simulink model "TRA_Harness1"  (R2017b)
settings: Solver=FixedStepDiscrete  StartTime=0.0  StopTime=16  FixedStep=0.01  RelTol=1e-3  EnableMultiTasking=on
undefined symbols (not defined in the file): sigbuilder_block
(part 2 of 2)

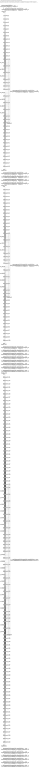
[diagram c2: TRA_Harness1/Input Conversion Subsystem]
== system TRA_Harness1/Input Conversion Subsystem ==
  note: This subsystem has been inserted by Simulink to adapt the output of the source blocks to the interface required by the harnessed component. Modifying the contents of this subsystem may result in compilation and simulation failure.
  Inport_1 : Inport
  Inport_2 : Inport  Port=2
  Inport_3 : Inport  Port=3
  Inport_4 : Inport  Port=4
  Inport_5 : Inport  Port=5
  Inport_6 : Inport  Port=6
  Inport_7 : Inport  Port=7
  Inport_8 : Inport  Port=8
  Inport_9 : Inport  Port=9
  Inport_10 : Inport  Port=10
  Inport_11 : Inport  Port=11
  Inport_12 : Inport  Port=12
  Inport_13 : Inport  Port=13
  Inport_14 : Inport  Port=14
  Inport_15 : Inport  Port=15
  Inport_16 : Inport  Port=16
  Inport_17 : Inport  Port=17
  Inport_18 : Inport  Port=18
  Inport_19 : Inport  Port=19
  Inport_20 : Inport  Port=20
  Inport_21 : Inport  Port=21
  Inport_22 : Inport  Port=22
  Inport_23 : Inport  Port=23
  Inport_24 : Inport  Port=24
  Inport_25 : Inport  Port=25
  Inport_26 : Inport  Port=26
  Inport_27 : Inport  Port=27
  Inport_28 : Inport  Port=28
  Inport_29 : Inport  Port=29
  Inport_30 : Inport  Port=30
  Inport_31 : Inport  Port=31
  Inport_32 : Inport  Port=32
  Inport_33 : Inport  Port=33
  Inport_34 : Inport  Port=34
  Inport_35 : Inport  Port=35
  Inport_36 : Inport  Port=36
  Inport_37 : Inport  Port=37
  Inport_38 : Inport  Port=38
  Inport_39 : Inport  Port=39
  Inport_40 : Inport  Port=40
  Inport_41 : Inport  Port=41
  Inport_42 : Inport  Port=42
  Inport_43 : Inport  Port=43
  Inport_44 : Inport  Port=44
  Inport_45 : Inport  Port=45
  Inport_46 : Inport  Port=46
  Inport_47 : Inport  Port=47
  Inport_48 : Inport  Port=48
  Inport_49 : Inport  Port=49
  Inport_50 : Inport  Port=50
  Inport_51 : Inport  Port=51
  Inport_52 : Inport  Port=52
  Inport_53 : Inport  Port=53
  Inport_54 : Inport  Port=54
  Inport_55 : Inport  Port=55
  Inport_56 : Inport  Port=56
  Inport_57 : Inport  Port=57
  Inport_58 : Inport  Port=58
  Inport_59 : Inport  Port=59
  Inport_60 : Inport  Port=60
  Inport_61 : Inport  Port=61
  Inport_62 : Inport  Port=62
  Inport_63 : Inport  Port=63
  Inport_64 : Inport  Port=64
  Inport_65 : Inport  Port=65
  Inport_66 : Inport  Port=66
  Inport_67 : Inport  Port=67
  Inport_68 : Inport  Port=68
  Inport_69 : Inport  Port=69
  Inport_70 : Inport  Port=70
  Inport_71 : Inport  Port=71
  Inport_72 : Inport  Port=72
  Inport_73 : Inport  Port=73
  Inport_74 : Inport  Port=74
  Inport_75 : Inport  Port=75
  Inport_76 : Inport  Port=76
  Inport_77 : Inport  Port=77
  Inport_78 : Inport  Port=78
  Inport_79 : Inport  Port=79
  Inport_80 : Inport  Port=80
  Inport_81 : Inport  Port=81
  Inport_82 : Inport  Port=82
  Inport_83 : Inport  Port=83
  Inport_84 : Inport  Port=84
  Inport_85 : Inport  Port=85
  Inport_86 : Inport  Port=86
  Inport_87 : Inport  Port=87
  Inport_88 : Inport  Port=88
  Inport_89 : Inport  Port=89
  Inport_90 : Inport  Port=90
  Inport_91 : Inport  Port=91
  Inport_92 : Inport  Port=92
  Inport_93 : Inport  Port=93
  Inport_94 : Inport  Port=94
  Inport_95 : Inport  Port=95
  Inport_96 : Inport  Port=96
  Inport_97 : Inport  Port=97
  Inport_98 : Inport  Port=98
  Inport_99 : Inport  Port=99
  Inport_100 : Inport  Port=100
  Inport_101 : Inport  Port=101
  Inport_102 : Inport  Port=102
  Inport_103 : Inport  Port=103
  Inport_104 : Inport  Port=104
  Inport_105 : Inport  Port=105
  Inport_106 : Inport  Port=106
  Inport_107 : Inport  Port=107
  Inport_108 : Inport  Port=108
  Inport_109 : Inport  Port=109
  Inport_110 : Inport  Port=110
  Inport_111 : Inport  Port=111
  Inport_112 : Inport  Port=112
  Inport_113 : Inport  Port=113
  Inport_114 : Inport  Port=114
  Inport_115 : Inport  Port=115
  Inport_116 : Inport  Port=116
  Inport_117 : Inport  Port=117
  Inport_118 : Inport  Port=118
  Inport_119 : Inport  Port=119
  Inport_120 : Inport  Port=120
  Inport_121 : Inport  Port=121
  Inport_122 : Inport  Port=122
  Inport_123 : Inport  Port=123
  Inport_124 : Inport  Port=124
  Inport_125 : Inport  Port=125
  Inport_126 : Inport  Port=126
  Inport_127 : Inport  Port=127
  Inport_128 : Inport  Port=128
  Inport_129 : Inport  Port=129
  Inport_130 : Inport  Port=130
  Inport_131 : Inport  Port=131
  Inport_132 : Inport  Port=132
  Inport_133 : Inport  Port=133
  Inport_134 : Inport  Port=134
  Inport_135 : Inport  Port=135
  Inport_136 : Inport  Port=136
  Inport_137 : Inport  Port=137
  Inport_138 : Inport  Port=138
  Inport_139 : Inport  Port=139
  Inport_140 : Inport  Port=140
  Inport_141 : Inport  Port=141
  Inport_142 : Inport  Port=142
  Inport_143 : Inport  Port=143
  Inport_144 : Inport  Port=144
  Inport_145 : Inport  Port=145
  Inport_146 : Inport  Port=146
  Inport_147 : Inport  Port=147
  Inport_148 : Inport  Port=148
  Inport_149 : Inport  Port=149
  Inport_150 : Inport  Port=150
  Inport_151 : Inport  Port=151
  Inport_152 : Inport  Port=152
  Inport_153 : Inport  Port=153
  Inport_154 : Inport  Port=154
  Inport_155 : Inport  Port=155
  Inport_156 : Inport  Port=156
  Inport_157 : Inport  Port=157
  Inport_158 : Inport  Port=158
  Inport_159 : Inport  Port=159
  Inport_160 : Inport  Port=160
  Inport_161 : Inport  Port=161
  Inport_162 : Inport  Port=162
  Inport_163 : Inport  Port=163
  Inport_164 : Inport  Port=164
  Inport_165 : Inport  Port=165
  Inport_166 : Inport  Port=166
  Inport_167 : Inport  Port=167
  Inport_168 : Inport  Port=168
  Inport_169 : Inport  Port=169
  Inport_170 : Inport  Port=170
  Inport_171 : Inport  Port=171
  Inport_172 : Inport  Port=172
  Inport_173 : Inport  Port=173
  Inport_174 : Inport  Port=174
  Inport_175 : Inport  Port=175
  Inport_176 : Inport  Port=176
  Inport_177 : Inport  Port=177
  Inport_178 : Inport  Port=178
  Inport_179 : Inport  Port=179
  Inport_180 : Inport  Port=180
  Inport_181 : Inport  Port=181
  Inport_182 : Inport  Port=182
  Inport_183 : Inport  Port=183
  Inport_184 : Inport  Port=184
  Inport_185 : Inport  Port=185
  Inport_186 : Inport  Port=186
  Inport_187 : Inport  Port=187
  Inport_188 : Inport  Port=188
  Inport_189 : Inport  Port=189
  Inport_190 : Inport  Port=190
  Inport_191 : Inport  Port=191
  Inport_192 : Inport  Port=192
  Inport_193 : Inport  Port=193
  Inport_194 : Inport  Port=194
  Inport_195 : Inport  Port=195
  Inport_196 : Inport  Port=196
  Inport_197 : Inport  Port=197
  Inport_198 : Inport  Port=198
  Inport_199 : Inport  Port=199
  Inport_200 : Inport  Port=200
  Inport_201 : Inport  Port=201
  Inport_202 : Inport  Port=202
  Inport_203 : Inport  Port=203
  Inport_204 : Inport  Port=204
  Inport_205 : Inport  Port=205
  Inport_206 : Inport  Port=206
  Inport_207 : Inport  Port=207
  Inport_208 : Inport  Port=208
  Inport_209 : Inport  Port=209
  Inport_210 : Inport  Port=210
  Inport_211 : Inport  Port=211
  Inport_212 : Inport  Port=212
  Inport_213 : Inport  Port=213
  Inport_214 : Inport  Port=214
  Inport_215 : Inport  Port=215
  Inport_216 : Inport  Port=216
  Inport_217 : Inport  Port=217
  Inport_218 : Inport  Port=218
  Inport_219 : Inport  Port=219
  Inport_220 : Inport  Port=220
  Inport_221 : Inport  Port=221
  Inport_222 : Inport  Port=222
  Inport_223 : Inport  Port=223
  Inport_224 : Inport  Port=224
  Inport_225 : Inport  Port=225
  Inport_226 : Inport  Port=226
  Inport_227 : Inport  Port=227
  Concat_1 : Concatenate  NumInputs=48
  Concat_2 : Concatenate  NumInputs=48
  Concat_3 : Concatenate  NumInputs=112
  Data_Conversion_{1..2,4,6..8,24} (7 alike) : DataTypeConversion  OutDataTypeStr=single
  Data_Conversion_{5,10..11,20,23} (5 alike) : DataTypeConversion  OutDataTypeStr=uint8
  Data_Conversion_{12,14..17,21} (6 alike) : DataTypeConversion  OutDataTypeStr=boolean
  Data_Conversion_13 : DataTypeConversion  OutDataTypeStr=uint32
  Data_Conversion_18 : DataTypeConversion  OutDataTypeStr=uint16
  Data_Conversion_19 : Reshape  OutputDimensionality=Customize  OutputDimensions=[112]
  Data_Conversion_22 : DataTypeConversion  OutDataTypeStr=uint16
  Data_Conversion_25 : DataTypeConversion  OutDataTypeStr=uint16
  Data_Conversion_3 : Reshape  OutputDimensionality=Customize  OutputDimensions=[48]
  Data_Conversion_9 : Reshape  OutputDimensionality=Customize  OutputDimensions=[48]
  RateTs_{1..22} (22 alike) : RateTransition
  SigSpec_1 : SignalSpecification
  SigSpec_10 : SignalSpecification  OutDataTypeStr=uint8  Unit=enum  Dimensions=[1]
  SigSpec_{11,13..16,19} (6 alike) : SignalSpecification  OutDataTypeStr=boolean  Unit=flag  Dimensions=[1]
  SigSpec_12 : SignalSpecification  OutDataTypeStr=uint32  Unit=min  Dimensions=[1]
  SigSpec_17 : SignalSpecification  OutDataTypeStr=uint16  Unit=mV  Dimensions=[112]
  SigSpec_18 : SignalSpecification  OutDataTypeStr=uint8  Unit=enum  Dimensions=[1]
  SigSpec_{2,4,6..7} (4 alike) : SignalSpecification  OutDataTypeStr=single  Unit=C  Dimensions=[1]
  SigSpec_20 : SignalSpecification  OutDataTypeStr=uint16  Unit=mV  Dimensions=[1]
  SigSpec_21 : SignalSpecification  OutDataTypeStr=uint8  Unit=numb  Dimensions=[1]
  SigSpec_22 : SignalSpecification  OutDataTypeStr=single  Unit=A  Dimensions=[1]
  SigSpec_23 : SignalSpecification  OutDataTypeStr=uint16  Unit=enum  Dimensions=[1]
  SigSpec_3 : SignalSpecification  OutDataTypeStr=single  Unit=C  Dimensions=[48]
  SigSpec_5 : SignalSpecification  OutDataTypeStr=uint8  Unit=numb  Dimensions=[1]
  SigSpec_8 : SignalSpecification  OutDataTypeStr=single  Unit=C  Dimensions=[48]
  SigSpec_9 : SignalSpecification  OutDataTypeStr=uint8  Unit=numb  Dimensions=[1]
  Outport_1 : Outport
  Outport_2 : Outport  Port=2
  Outport_3 : Outport  Port=3
  Outport_4 : Outport  Port=4
  Outport_5 : Outport  Port=5
  Outport_6 : Outport  Port=6
  Outport_7 : Outport  Port=7
  Outport_8 : Outport  Port=8
  Outport_9 : Outport  Port=9
  Outport_10 : Outport  Port=10
  Outport_11 : Outport  Port=11
  Outport_12 : Outport  Port=12
  Outport_13 : Outport  Port=13
  Outport_14 : Outport  Port=14
  Outport_15 : Outport  Port=15
  Outport_16 : Outport  Port=16
  Outport_17 : Outport  Port=17
  Outport_18 : Outport  Port=18
  Outport_19 : Outport  Port=19
  Outport_20 : Outport  Port=20
  Outport_21 : Outport  Port=21
  Outport_22 : Outport  Port=22
  Outport_23 : Outport  Port=23
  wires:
  SigSpec_1/1 -> Outport_1/1
  [send_fcn1] -> SigSpec_1/1
  SigSpec_2/1 -> Outport_2/1
  RateTs_1/1 -> SigSpec_2/1
  Data_Conversion_1/1 -> RateTs_1/1
  Inport_1/1 -> Data_Conversion_1/1
  SigSpec_3/1 -> Outport_3/1
  RateTs_2/1 -> SigSpec_3/1
  Data_Conversion_2/1 -> RateTs_2/1
  Data_Conversion_3/1 -> Data_Conversion_2/1
  Concat_1/1 -> Data_Conversion_3/1
  Inport_2/1 -> Concat_1/1
  Inport_3/1 -> Concat_1/2
  Inport_4/1 -> Concat_1/3
  Inport_5/1 -> Concat_1/4
  Inport_6/1 -> Concat_1/5
  Inport_7/1 -> Concat_1/6
  Inport_8/1 -> Concat_1/7
  Inport_9/1 -> Concat_1/8
  Inport_10/1 -> Concat_1/9
  Inport_11/1 -> Concat_1/10
  Inport_12/1 -> Concat_1/11
  Inport_13/1 -> Concat_1/12
  Inport_14/1 -> Concat_1/13
  Inport_15/1 -> Concat_1/14
  Inport_16/1 -> Concat_1/15
  Inport_17/1 -> Concat_1/16
  Inport_18/1 -> Concat_1/17
  Inport_19/1 -> Concat_1/18
  Inport_20/1 -> Concat_1/19
  Inport_21/1 -> Concat_1/20
  Inport_22/1 -> Concat_1/21
  Inport_23/1 -> Concat_1/22
  Inport_24/1 -> Concat_1/23
  Inport_25/1 -> Concat_1/24
  Inport_26/1 -> Concat_1/25
  Inport_27/1 -> Concat_1/26
  Inport_28/1 -> Concat_1/27
  Inport_29/1 -> Concat_1/28
  Inport_30/1 -> Concat_1/29
  Inport_31/1 -> Concat_1/30
  Inport_32/1 -> Concat_1/31
  Inport_33/1 -> Concat_1/32
  Inport_34/1 -> Concat_1/33
  Inport_35/1 -> Concat_1/34
  Inport_36/1 -> Concat_1/35
  Inport_37/1 -> Concat_1/36
  Inport_38/1 -> Concat_1/37
  Inport_39/1 -> Concat_1/38
  Inport_40/1 -> Concat_1/39
  Inport_41/1 -> Concat_1/40
  Inport_42/1 -> Concat_1/41
  Inport_43/1 -> Concat_1/42
  Inport_44/1 -> Concat_1/43
  Inport_45/1 -> Concat_1/44
  Inport_46/1 -> Concat_1/45
  Inport_47/1 -> Concat_1/46
  Inport_48/1 -> Concat_1/47
  Inport_49/1 -> Concat_1/48
  SigSpec_4/1 -> Outport_4/1
  RateTs_3/1 -> SigSpec_4/1
  Data_Conversion_4/1 -> RateTs_3/1
  Inport_50/1 -> Data_Conversion_4/1
  SigSpec_5/1 -> Outport_5/1
  RateTs_4/1 -> SigSpec_5/1
  Data_Conversion_5/1 -> RateTs_4/1
  Inport_51/1 -> Data_Conversion_5/1
  SigSpec_6/1 -> Outport_6/1
  RateTs_5/1 -> SigSpec_6/1
  Data_Conversion_6/1 -> RateTs_5/1
  Inport_52/1 -> Data_Conversion_6/1
  SigSpec_7/1 -> Outport_7/1
  RateTs_6/1 -> SigSpec_7/1
  Data_Conversion_7/1 -> RateTs_6/1
  Inport_53/1 -> Data_Conversion_7/1
  SigSpec_8/1 -> Outport_8/1
  RateTs_7/1 -> SigSpec_8/1
  Data_Conversion_8/1 -> RateTs_7/1
  Data_Conversion_9/1 -> Data_Conversion_8/1
  Concat_2/1 -> Data_Conversion_9/1
  Inport_54/1 -> Concat_2/1
  Inport_55/1 -> Concat_2/2
  Inport_56/1 -> Concat_2/3
  Inport_57/1 -> Concat_2/4
  Inport_58/1 -> Concat_2/5
  Inport_59/1 -> Concat_2/6
  Inport_60/1 -> Concat_2/7
  Inport_61/1 -> Concat_2/8
  Inport_62/1 -> Concat_2/9
  Inport_63/1 -> Concat_2/10
  Inport_64/1 -> Concat_2/11
  Inport_65/1 -> Concat_2/12
  Inport_66/1 -> Concat_2/13
  Inport_67/1 -> Concat_2/14
  Inport_68/1 -> Concat_2/15
  Inport_69/1 -> Concat_2/16
  Inport_70/1 -> Concat_2/17
  Inport_71/1 -> Concat_2/18
  Inport_72/1 -> Concat_2/19
  Inport_73/1 -> Concat_2/20
  Inport_74/1 -> Concat_2/21
  Inport_75/1 -> Concat_2/22
  Inport_76/1 -> Concat_2/23
  Inport_77/1 -> Concat_2/24
  Inport_78/1 -> Concat_2/25
  Inport_79/1 -> Concat_2/26
  Inport_80/1 -> Concat_2/27
  Inport_81/1 -> Concat_2/28
  Inport_82/1 -> Concat_2/29
  Inport_83/1 -> Concat_2/30
  Inport_84/1 -> Concat_2/31
  Inport_85/1 -> Concat_2/32
  Inport_86/1 -> Concat_2/33
  Inport_87/1 -> Concat_2/34
  Inport_88/1 -> Concat_2/35
  Inport_89/1 -> Concat_2/36
  Inport_90/1 -> Concat_2/37
  Inport_91/1 -> Concat_2/38
  Inport_92/1 -> Concat_2/39
  Inport_93/1 -> Concat_2/40
  Inport_94/1 -> Concat_2/41
  Inport_95/1 -> Concat_2/42
  Inport_96/1 -> Concat_2/43
  Inport_97/1 -> Concat_2/44
  Inport_98/1 -> Concat_2/45
  Inport_99/1 -> Concat_2/46
  Inport_100/1 -> Concat_2/47
  Inport_101/1 -> Concat_2/48
  SigSpec_9/1 -> Outport_9/1
  RateTs_8/1 -> SigSpec_9/1
  Data_Conversion_10/1 -> RateTs_8/1
  Inport_102/1 -> Data_Conversion_10/1
  SigSpec_10/1 -> Outport_10/1
  RateTs_9/1 -> SigSpec_10/1
  Data_Conversion_11/1 -> RateTs_9/1
  Inport_103/1 -> Data_Conversion_11/1
  SigSpec_11/1 -> Outport_11/1
  RateTs_10/1 -> SigSpec_11/1
  Data_Conversion_12/1 -> RateTs_10/1
  Inport_104/1 -> Data_Conversion_12/1
  SigSpec_12/1 -> Outport_12/1
  RateTs_11/1 -> SigSpec_12/1
  Data_Conversion_13/1 -> RateTs_11/1
  Inport_105/1 -> Data_Conversion_13/1
  SigSpec_13/1 -> Outport_13/1
  RateTs_12/1 -> SigSpec_13/1
  Data_Conversion_14/1 -> RateTs_12/1
  Inport_106/1 -> Data_Conversion_14/1
  SigSpec_14/1 -> Outport_14/1
  RateTs_13/1 -> SigSpec_14/1
  Data_Conversion_15/1 -> RateTs_13/1
  Inport_107/1 -> Data_Conversion_15/1
  SigSpec_15/1 -> Outport_15/1
  RateTs_14/1 -> SigSpec_15/1
  Data_Conversion_16/1 -> RateTs_14/1
  Inport_108/1 -> Data_Conversion_16/1
  SigSpec_16/1 -> Outport_16/1
  RateTs_15/1 -> SigSpec_16/1
  Data_Conversion_17/1 -> RateTs_15/1
  Inport_109/1 -> Data_Conversion_17/1
  SigSpec_17/1 -> Outport_17/1
  RateTs_16/1 -> SigSpec_17/1
  Data_Conversion_18/1 -> RateTs_16/1
  Data_Conversion_19/1 -> Data_Conversion_18/1
  Concat_3/1 -> Data_Conversion_19/1
  Inport_110/1 -> Concat_3/1
  Inport_111/1 -> Concat_3/2
  Inport_112/1 -> Concat_3/3
  Inport_113/1 -> Concat_3/4
  Inport_114/1 -> Concat_3/5
  Inport_115/1 -> Concat_3/6
  Inport_116/1 -> Concat_3/7
  Inport_117/1 -> Concat_3/8
  Inport_118/1 -> Concat_3/9
  Inport_119/1 -> Concat_3/10
  Inport_120/1 -> Concat_3/11
  Inport_121/1 -> Concat_3/12
  Inport_122/1 -> Concat_3/13
  Inport_123/1 -> Concat_3/14
  Inport_124/1 -> Concat_3/15
  Inport_125/1 -> Concat_3/16
  Inport_126/1 -> Concat_3/17
  Inport_127/1 -> Concat_3/18
  Inport_128/1 -> Concat_3/19
  Inport_129/1 -> Concat_3/20
  Inport_130/1 -> Concat_3/21
  Inport_131/1 -> Concat_3/22
  Inport_132/1 -> Concat_3/23
  Inport_133/1 -> Concat_3/24
  Inport_134/1 -> Concat_3/25
  Inport_135/1 -> Concat_3/26
  Inport_136/1 -> Concat_3/27
  Inport_137/1 -> Concat_3/28
  Inport_138/1 -> Concat_3/29
  Inport_139/1 -> Concat_3/30
  Inport_140/1 -> Concat_3/31
  Inport_141/1 -> Concat_3/32
  Inport_142/1 -> Concat_3/33
  Inport_143/1 -> Concat_3/34
  Inport_144/1 -> Concat_3/35
  Inport_145/1 -> Concat_3/36
  Inport_146/1 -> Concat_3/37
  Inport_147/1 -> Concat_3/38
  Inport_148/1 -> Concat_3/39
  Inport_149/1 -> Concat_3/40
  Inport_150/1 -> Concat_3/41
  Inport_151/1 -> Concat_3/42
  Inport_152/1 -> Concat_3/43
  Inport_153/1 -> Concat_3/44
  Inport_154/1 -> Concat_3/45
  Inport_155/1 -> Concat_3/46
  Inport_156/1 -> Concat_3/47
  Inport_157/1 -> Concat_3/48
  Inport_158/1 -> Concat_3/49
  Inport_159/1 -> Concat_3/50
  Inport_160/1 -> Concat_3/51
  Inport_161/1 -> Concat_3/52
  Inport_162/1 -> Concat_3/53
  Inport_163/1 -> Concat_3/54
  Inport_164/1 -> Concat_3/55
  Inport_165/1 -> Concat_3/56
  Inport_166/1 -> Concat_3/57
  Inport_167/1 -> Concat_3/58
  Inport_168/1 -> Concat_3/59
  Inport_169/1 -> Concat_3/60
  Inport_170/1 -> Concat_3/61
  Inport_171/1 -> Concat_3/62
  Inport_172/1 -> Concat_3/63
  Inport_173/1 -> Concat_3/64
  Inport_174/1 -> Concat_3/65
  Inport_175/1 -> Concat_3/66
  Inport_176/1 -> Concat_3/67
  Inport_177/1 -> Concat_3/68
  Inport_178/1 -> Concat_3/69
  Inport_179/1 -> Concat_3/70
  Inport_180/1 -> Concat_3/71
  Inport_181/1 -> Concat_3/72
  Inport_182/1 -> Concat_3/73
  Inport_183/1 -> Concat_3/74
  Inport_184/1 -> Concat_3/75
  Inport_185/1 -> Concat_3/76
  Inport_186/1 -> Concat_3/77
  Inport_187/1 -> Concat_3/78
  Inport_188/1 -> Concat_3/79
  Inport_189/1 -> Concat_3/80
  Inport_190/1 -> Concat_3/81
  Inport_191/1 -> Concat_3/82
  Inport_192/1 -> Concat_3/83
  Inport_193/1 -> Concat_3/84
  Inport_194/1 -> Concat_3/85
  Inport_195/1 -> Concat_3/86
  Inport_196/1 -> Concat_3/87
  Inport_197/1 -> Concat_3/88
  Inport_198/1 -> Concat_3/89
  Inport_199/1 -> Concat_3/90
  Inport_200/1 -> Concat_3/91
  Inport_201/1 -> Concat_3/92
  Inport_202/1 -> Concat_3/93
  Inport_203/1 -> Concat_3/94
  Inport_204/1 -> Concat_3/95
  Inport_205/1 -> Concat_3/96
  Inport_206/1 -> Concat_3/97
  Inport_207/1 -> Concat_3/98
  Inport_208/1 -> Concat_3/99
  Inport_209/1 -> Concat_3/100
  Inport_210/1 -> Concat_3/101
  Inport_211/1 -> Concat_3/102
  Inport_212/1 -> Concat_3/103
  Inport_213/1 -> Concat_3/104
  Inport_214/1 -> Concat_3/105
  Inport_215/1 -> Concat_3/106
  Inport_216/1 -> Concat_3/107
  Inport_217/1 -> Concat_3/108
  Inport_218/1 -> Concat_3/109
  Inport_219/1 -> Concat_3/110
  Inport_220/1 -> Concat_3/111
  Inport_221/1 -> Concat_3/112
  SigSpec_18/1 -> Outport_18/1
  RateTs_17/1 -> SigSpec_18/1
  Data_Conversion_20/1 -> RateTs_17/1
  Inport_222/1 -> Data_Conversion_20/1
  SigSpec_19/1 -> Outport_19/1
  RateTs_18/1 -> SigSpec_19/1
  Data_Conversion_21/1 -> RateTs_18/1
  Inport_223/1 -> Data_Conversion_21/1
  SigSpec_20/1 -> Outport_20/1
  RateTs_19/1 -> SigSpec_20/1
  Data_Conversion_22/1 -> RateTs_19/1
  Inport_224/1 -> Data_Conversion_22/1
  SigSpec_21/1 -> Outport_21/1
  RateTs_20/1 -> SigSpec_21/1
  Data_Conversion_23/1 -> RateTs_20/1
  Inport_225/1 -> Data_Conversion_23/1
  SigSpec_22/1 -> Outport_22/1
  RateTs_21/1 -> SigSpec_22/1
  Data_Conversion_24/1 -> RateTs_21/1
  Inport_226/1 -> Data_Conversion_24/1
  SigSpec_23/1 -> Outport_23/1
  RateTs_22/1 -> SigSpec_23/1
  Data_Conversion_25/1 -> RateTs_22/1
  Inport_227/1 -> Data_Conversion_25/1

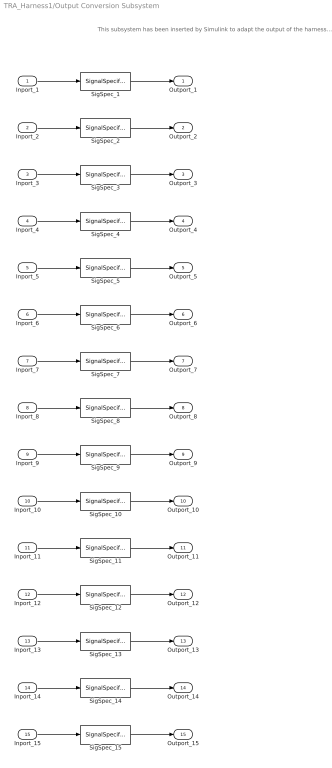
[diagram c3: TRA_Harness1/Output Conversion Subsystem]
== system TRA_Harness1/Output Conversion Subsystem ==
  note: This subsystem has been inserted by Simulink to adapt the output of the harnessed component to the interface required by the sink blocks. Modifying the contents of this subsystem may result in compilation and simulation failure.
  Inport_1 : Inport
  Inport_2 : Inport  Port=2
  Inport_3 : Inport  Port=3
  Inport_4 : Inport  Port=4
  Inport_5 : Inport  Port=5
  Inport_6 : Inport  Port=6
  Inport_7 : Inport  Port=7
  Inport_8 : Inport  Port=8
  Inport_9 : Inport  Port=9
  Inport_10 : Inport  Port=10
  Inport_11 : Inport  Port=11
  Inport_12 : Inport  Port=12
  Inport_13 : Inport  Port=13
  Inport_14 : Inport  Port=14
  Inport_15 : Inport  Port=15
  SigSpec_{1..3,8..9,15} (6 alike) : SignalSpecification  OutDataTypeStr=boolean  Unit=flag  Dimensions=[1]
  SigSpec_10 : SignalSpecification  OutDataTypeStr=uint8  Unit=enum  Dimensions=[1]
  SigSpec_{11..14} (4 alike) : SignalSpecification  OutDataTypeStr=uint16  Unit=mV  Dimensions=[1]
  SigSpec_4 : SignalSpecification  OutDataTypeStr=uint8  Unit=numb  Dimensions=[1]
  SigSpec_5 : SignalSpecification  OutDataTypeStr=uint16  Unit=min  Dimensions=[1]
  SigSpec_6 : SignalSpecification  OutDataTypeStr=uint32  Unit=min  Dimensions=[1]
  SigSpec_7 : SignalSpecification  OutDataTypeStr=single  Unit=pct  Dimensions=[1]
  Outport_1 : Outport
  Outport_2 : Outport  Port=2
  Outport_3 : Outport  Port=3
  Outport_4 : Outport  Port=4
  Outport_5 : Outport  Port=5
  Outport_6 : Outport  Port=6
  Outport_7 : Outport  Port=7
  Outport_8 : Outport  Port=8
  Outport_9 : Outport  Port=9
  Outport_10 : Outport  Port=10
  Outport_11 : Outport  Port=11
  Outport_12 : Outport  Port=12
  Outport_13 : Outport  Port=13
  Outport_14 : Outport  Port=14
  Outport_15 : Outport  Port=15
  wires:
  Inport_1/1 -> SigSpec_1/1
  SigSpec_1/1 -> Outport_1/1
  Inport_2/1 -> SigSpec_2/1
  SigSpec_2/1 -> Outport_2/1
  Inport_3/1 -> SigSpec_3/1
  SigSpec_3/1 -> Outport_3/1
  Inport_4/1 -> SigSpec_4/1
  SigSpec_4/1 -> Outport_4/1
  Inport_5/1 -> SigSpec_5/1
  SigSpec_5/1 -> Outport_5/1
  Inport_6/1 -> SigSpec_6/1
  SigSpec_6/1 -> Outport_6/1
  Inport_7/1 -> SigSpec_7/1
  SigSpec_7/1 -> Outport_7/1
  Inport_8/1 -> SigSpec_8/1
  SigSpec_8/1 -> Outport_8/1
  Inport_9/1 -> SigSpec_9/1
  SigSpec_9/1 -> Outport_9/1
  Inport_10/1 -> SigSpec_10/1
  SigSpec_10/1 -> Outport_10/1
  Inport_11/1 -> SigSpec_11/1
  SigSpec_11/1 -> Outport_11/1
  Inport_12/1 -> SigSpec_12/1
  SigSpec_12/1 -> Outport_12/1
  Inport_13/1 -> SigSpec_13/1
  SigSpec_13/1 -> Outport_13/1
  Inport_14/1 -> SigSpec_14/1
  SigSpec_14/1 -> Outport_14/1
  Inport_15/1 -> SigSpec_15/1
  SigSpec_15/1 -> Outport_15/1

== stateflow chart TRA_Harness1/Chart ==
  (default) -> (junction 1)
  (junction 1) -> (junction 3) : {Run10ms}
  events: output FUNCTION_CALL_EVENT

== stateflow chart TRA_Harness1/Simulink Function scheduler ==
  state Run
  state AsyncFunctionCalls
    % Call Asynchronous FunctionCall Subsystems.
    %
    %% Schedule function-call outputs.
    %% Modify this code to change function-call order.
    send(TRA_ThemRunAway_10ms)
  (default) -> Run
  events: output FUNCTION_CALL_EVENT
